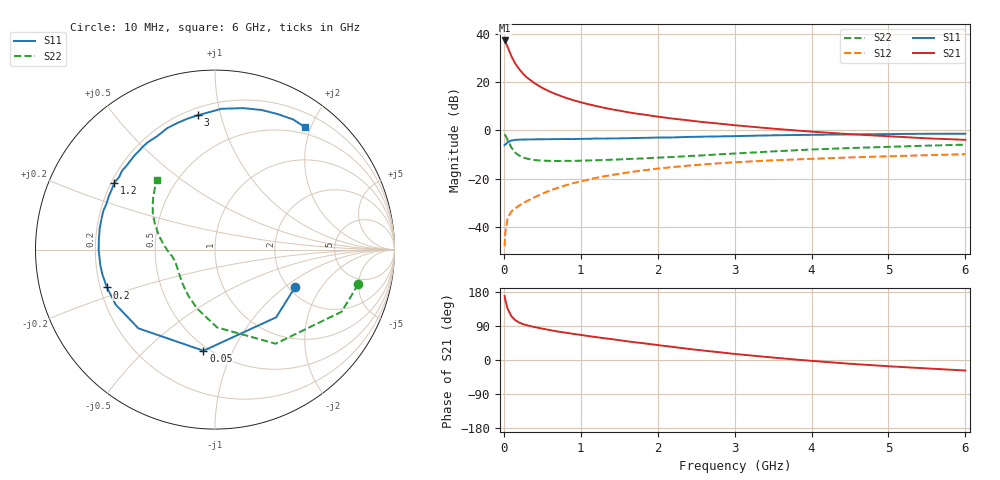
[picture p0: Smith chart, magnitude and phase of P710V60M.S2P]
! SIEMENS Small Signal Semiconductors
! BFP196
! Si NPN RF Bipolar Junction Transistor in SOT143
! VCE = 10 V  IC = 60 mA
! Common Emitter S-Parameters:  May  1996
# GHz  S  MA  R  50
!  f  S11  S21  S12  S22
! GHz  MAG  ANG  MAG  ANG  MAG  ANG  MAG  ANG
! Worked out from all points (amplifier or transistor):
!   36 points, 10 MHz to 6 GHz, reference 50 ohm
!   highest |S21| = 37.1 dB at 10 MHz (marker M1)
!   |S21| within 3 dB of that: start of sweep to 53.18 MHz
!   unconditionally stable (mu >= 1): 492 MHz to 4.534 GHz
!   at 250 MHz: K = 0.80, MSG = 26.8 dB, |S12| = -30.2 dB
!   at 1.4 GHz: K = 1.08, MAG = 11.8 dB, |S12| = -18.5 dB
!   at 6 GHz: K = 0.98, MSG = 3.0 dB, |S12| = -9.9 dB
!   S11 on the Smith chart (normalised r, x): 10 MHz: 2.16, -1.19; 50 MHz: 0.47, -0.78; 200 MHz: 0.23, -0.16; 1.2 GHz: 0.21, +0.29; 3 GHz: 0.25, +0.85; 6 GHz: 0.40, +1.91
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0.01  0.4927 -25.2  71.88 168.6  0.004 72.3  0.8218 -13.6
0.02  0.5084 -47.9  67.17 157.7  0.0077 65.8  0.7851 -26.2
0.05  0.5672 -96.5  52.35 134.8  0.0153 54.6  0.6237 -57.2
0.1  0.6119 -134.2  33.55 114.8  0.0211 47.4  0.4336 -88.5
0.15  0.6326 -151.0  23.76 104.8  0.0245 46.8  0.3431 -106.9
0.2  0.6379 -160.7  18.32 98.8  0.0276 49.0  0.2985 -119.4
0.25  0.6426 -167.7  14.74 94.6  0.031 50.7  0.272 -128.9
0.3  0.6449 -172.4  12.34 91.6  0.0342 54.1  0.2587 -135.3
0.4  0.6481 180.0  9.374 86.9  0.0411 57.2  0.2421 -145.2
0.5  0.6497 174.7  7.5 82.8  0.0487 59.1  0.2351 -151.7
0.6  0.6532 169.6  6.266 78.9  0.0566 60.0  0.2321 -156.2
0.7  0.6549 165.0  5.388 75.2  0.0641 60.5  0.2314 -159.5
0.9  0.6565 157.3  4.193 69.1  0.0803 59.9  0.2324 -164.6
1.1  0.6652 150.0  3.447 63.2  0.0954 58.3  0.2372 -168.0
1.2  0.6732 146.3  3.164 60.4  0.1034 57.5  0.2399 -169.9
1.6  0.6837 133.6  2.375 49.5  0.1328 52.4  0.2535 -175.3
2.2  0.7097 116.9  1.736 34.4  0.1732 44.0  0.2801 176.5
3  0.7544 97.2  1.27 16.0  0.2175 32.4  0.3298 164.1
3.5  0.7853 87.4  1.077 6.4  0.2384 25.5  0.3648 156.7
4.5  0.8205 71.4  0.828 -9.9  0.2738 13.9  0.4276 144.3
5.5  0.8458 59.0  0.68 -22.2  0.3044 3.5  0.4797 134.3
6  0.8469 53.6  0.633 -27.8  0.3192 -2.1  0.5037 129.5
